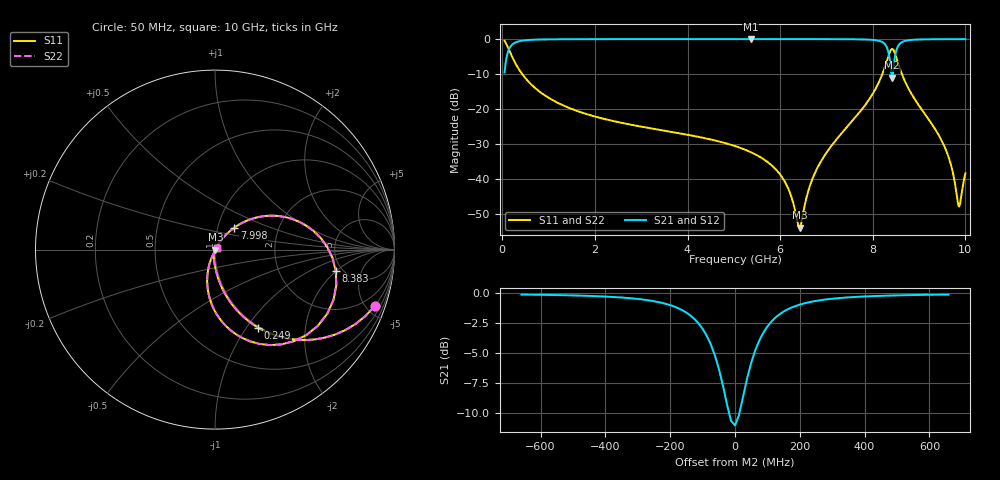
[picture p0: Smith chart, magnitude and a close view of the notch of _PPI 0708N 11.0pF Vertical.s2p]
! S-Parameter data specifications (vertical orientation):
! Substrate: 40-mil Rogers 3003C, Substrate thickness, H=1.016mm, Dielectric constant, Er=3, Conductor thickness, T_mtl=0.043mm, Loss Tangent, Tand=0.003
! PCB Mounting Pad Footprint: Pad width, PadW=2.54mm , Pad length, PadL=0.51mm , Pad gap, PadG (edge-to-edge)=0.71mm , Reference planes=1.73mm apart
! Created Tue Jan 16 08:47:09 2018
# GHz S MA R 50
! 2 Port Network Data from SP1.SP block
! freq  magS11  angS11  magS21  angS21  magS12  angS12  magS22  angS22
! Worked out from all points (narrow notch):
!   801 points, 50 MHz to 10 GHz, reference 50 ohm
!   highest |S21| = -0.02 dB at 5.361 GHz (marker M1); lowest = -11.1 dB at 8.42 GHz (marker M2)
!   notch at M2: 11.0 dB deep, 111 MHz wide at half that depth
!   lowest |S11| = -54.0 dB at 6.418 GHz (marker M3), VSWR 1.00, Z = 50.2 - j0.0785 ohm
!   |S11| at or under -10 dB: 428 MHz to 8.208 GHz (7.78 GHz wide, 180 % of centre); 8.629 GHz to end of sweep
!   |S22| runs from -54.0 to -0.5 dB; largest |S21 - S12| = 0
!   S11 on the Smith chart (normalised r, x): 50 MHz: 0.98, -5.63; 249 MHz: 0.98, -1.13; 7.998 GHz: 1.20, +0.30; 8.383 GHz: 4.41, -1.95; 10 GHz: 1.02, +0.01
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0.05  0.9432 -19.6  0.3322 70.4  0.3322 70.4  0.9432 -19.6
0.249  0.4958 -61.1  0.8682 28.9  0.8682 28.9  0.4958 -61.1
0.79625  0.1785 -82.3  0.9835 7.5  0.9835 7.5  0.1785 -82.3
1.716625  0.08864 -90.5  0.9954 -0.9  0.9954 -0.9  0.08864 -90.5
3.370812  0.05048 -97.7  0.9977 -8.7  0.9977 -8.7  0.05048 -97.7
5.025  0.02938 -103.0  0.998 -15.6  0.998 -15.6  0.02938 -103.0
5.360812  0.02411 -103.6  0.9981 -17.0  0.9981 -17.0  0.02411 -103.6
6.032438  0.01073 -100.7  0.998 -20.0  0.998 -20.0  0.01073 -100.7
6.418  0.001998 -23.1  0.9977 -21.9  0.9977 -21.9  0.001998 -23.1
6.691625  0.009762 53.3  0.9974 -23.3  0.9974 -23.3  0.009762 53.3
7.027437  0.02508 58.3  0.9966 -25.3  0.9966 -25.3  0.02508 58.3
7.997562  0.1639 48.6  0.972 -36.4  0.972 -36.4  0.1639 48.6
8.196563  0.3029 36.8  0.9109 -45.1  0.9109 -45.1  0.3029 36.8
8.345812  0.592 6.3  0.6112 -61.3  0.6112 -61.3  0.592 6.3
8.383125  0.6831 -9.9  0.4116 -59.7  0.4116 -59.7  0.6831 -9.9
8.420438  0.7203 -29.7  0.2801 -24.9  0.2801 -24.9  0.7203 -29.7
8.495062  0.5798 -64.9  0.6334 4.2  0.6334 4.2  0.5798 -64.9
8.65675  0.2841 -95.3  0.9222 -12.8  0.9222 -12.8  0.2841 -95.3
9.539813  0.02979 -111.7  0.9948 -30.2  0.9948 -30.2  0.02979 -111.7
9.689063  0.01572 -106.2  0.9953 -31.5  0.9953 -31.5  0.01572 -106.2
9.85075  0.004147 -47.2  0.9956 -32.8  0.9956 -32.8  0.004147 -47.2
10  0.01196 36.6  0.9955 -34.0  0.9955 -34.0  0.01196 36.6
